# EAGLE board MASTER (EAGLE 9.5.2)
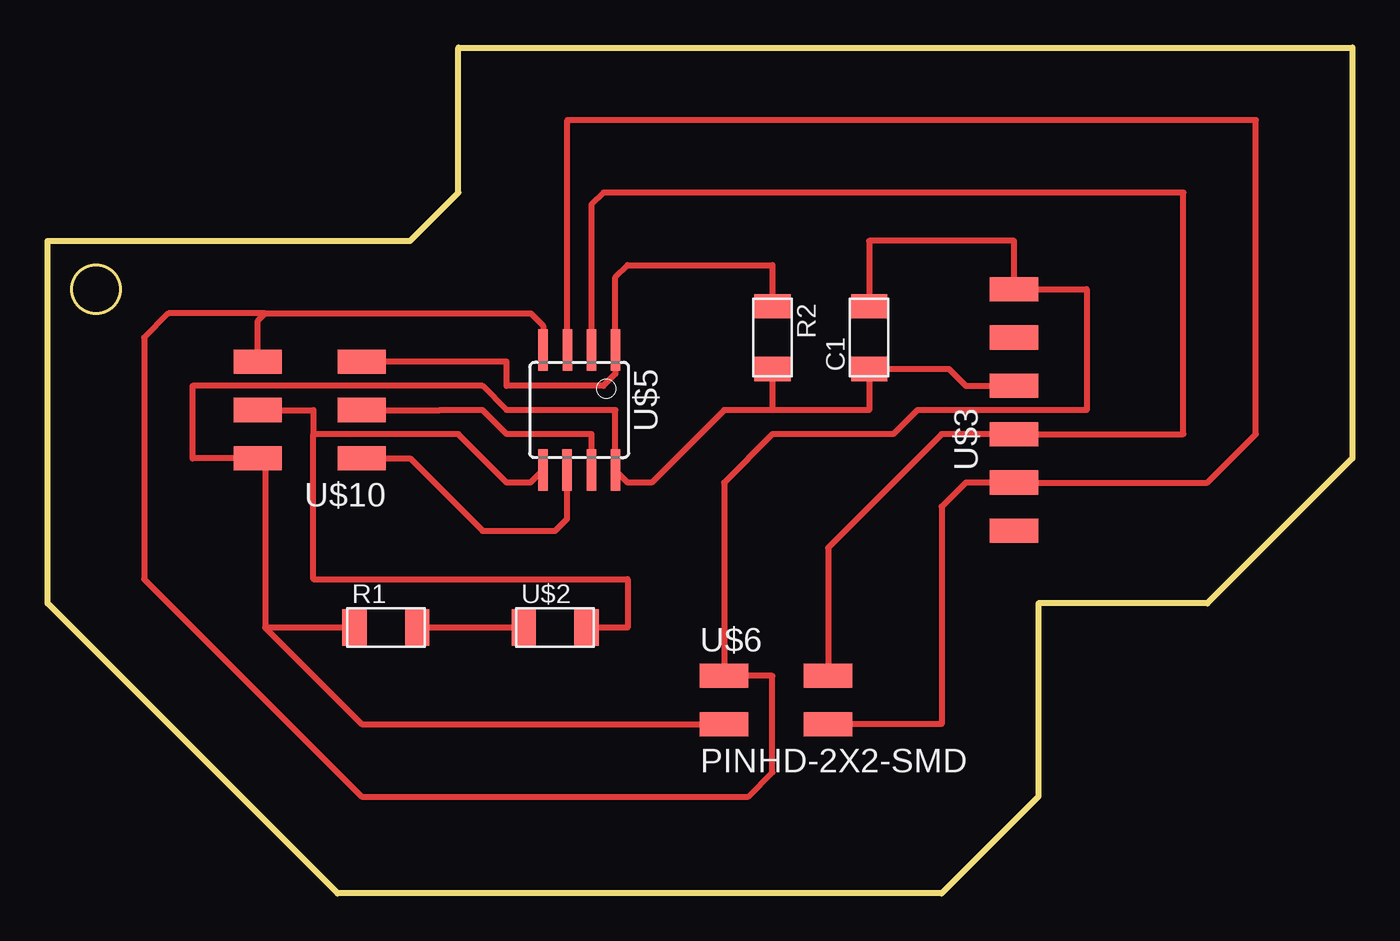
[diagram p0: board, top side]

Size 68.58 x 44.45 mm. Coordinates in mm from the lower left corner, seen from the top.
Outline: 0,34.29 19.05,34.29 21.59,36.83 21.59,44.45 68.58,44.45 68.58,22.86 60.96,15.24 52.07,15.24 52.07,5.08 46.99,0 15.24,0 0,15.24 0,34.29
Outline: circle at 2.54,31.75 radius 1.27
Copper layers (1*16): Top 0.035mm / dielectric 1.5mm / Bottom 0.035mm
Design rules "default": minimum track width 6mil, minimum drill 0.35mm, track to track 6mil, track to pad 6mil, pad to pad 6mil, via to via 6mil, smd to smd 6mil, copper to edge 40mil, drill to drill 6mil, minimum pad ring 10mil, minimum via ring 8mil, stop-mask expansion 4mil, vias tented up to drill 0mil, thermal gap 10mil

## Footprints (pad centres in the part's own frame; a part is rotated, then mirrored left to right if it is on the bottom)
C1206FAB = smd 1.27 x 1.905: 1 -1.651,0; 2 1.651,0
R1206FAB = smd 1.27 x 1.905: 1 -1.651,0; 2 1.651,0
LED1206FAB = smd 1.27 x 1.905: 1 -1.651,0; 2 1.651,0
1X06SMD = smd 2.54 x 1.27: 1 0,6.35; 2 0,3.81; 3 0,1.27; 4 0,-1.27; 5 0,-3.81; 6 0,-6.35
SOIC8 = smd 0.5 x 2.2: 1 -1.905,-3.154; 2 -0.645,-3.154; 3 0.625,-3.154; 4 1.895,-3.154; 5 1.905,3.154; 6 0.635,3.154; 7 -0.635,3.154; 8 -1.905,3.154
2X02SMD = smd 2.54 x 1.27: 1 -2.54,1.27; 2 2.92,1.27; 3 -2.54,-1.27; 4 2.92,-1.27
2X03SMD = smd 2.54 x 1.27: 1 -2.54,2.54; 2 2.92,2.54; 3 -2.54,0; 4 2.92,0; 5 -2.54,-2.54; 6 2.92,-2.54

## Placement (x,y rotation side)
C1  CAP-US1206FAB  [C1206FAB]  43.18,29.21 90 top
R1  [R1206FAB]  17.78,13.97 0 top
R2  [R1206FAB]  38.1,29.21 270 top
U$2  LEDFAB1206  [LED1206FAB]  26.67,13.97 0 top
U$3  FTDI-SMD-HEADER  [1X06SMD]  50.8,25.4 0 top
U$5  ATTINY45SI  [SOIC8]  27.94,25.4 180 top
U$6  PINHD-2X2-SMD  [2X02SMD]  38.1,10.16 0 top
U$10  AVRISPSMD  [2X03SMD]  13.97,25.4 180 top

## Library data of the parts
C1 R1 R2 U$2 U$3 U$5 U$6 U$10 = eagle_fab

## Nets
GND: C1.2 U$3.1 U$5.4 U$6.1 U$10.6
MISO: U$5.6 U$10.1
MOSI: U$2.2 U$5.5 U$10.4
N$2: R1.2 U$2.1
RST: R2.1 U$5.1 U$10.5
RXD: U$3.5 U$5.3 U$6.4
SCK: U$5.7 U$10.3
TXD: U$3.4 U$5.2 U$6.2
VCC: C1.1 R1.1 R2.2 U$3.3 U$5.8 U$6.3 U$10.2

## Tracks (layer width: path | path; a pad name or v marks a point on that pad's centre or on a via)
GND
  Top 0.152: 26.04,29.21 U$5.4
  Top 0.305: C1.2 43.18,34.29 50.8,34.29 U$3.1 54.61,31.75 54.61,25.4 45.72,25.4 44.45,24.13 38.1,24.13 35.56,21.59 U$6.1 38.1,11.43 38.1,6.35 36.83,5.08 16.51,5.08 5.08,16.51 5.08,29.21 6.35,30.48 11.43,30.48 | 11.43,30.48 25.4,30.48 26.04,29.83 26.04,29.21 | U$10.6 11.05,30.1 11.43,30.48
MISO
  Top 0.305: U$10.1 19.05,22.86 22.86,19.05 26.67,19.05 27.3,19.68 U$5.6
MOSI
  Top 0.305: U$10.4 13.97,25.4 13.97,24.13 | U$5.5 25.38,21.59 24.13,21.59 21.59,24.13 13.97,24.13 | 13.97,24.13 13.97,16.51 30.48,16.51 30.48,13.97 U$2.2
N$2
  Top 0.305: U$2.1 R1.2
RST
  Top 0.305: U$10.5 24.13,27.94 24.13,26.67 29.21,26.67 29.85,27.31 U$5.1 29.85,32.39 30.48,33.02 38.1,33.02 R2.1
RXD
  Top 0.152: 40.64,8.89 U$6.4
  Top 0.305: U$5.3 27.32,40.64 63.5,40.64 63.5,24.13 60.96,21.59 U$3.5 48.26,21.59 46.99,20.32 46.99,8.89 40.64,8.89
SCK
  Top 0.305: U$5.7 28.57,24.13 24.13,24.13 22.86,25.4 20.62,25.4 U$10.3
TXD
  Top 0.305: U$6.2 41.02,18.16 46.99,24.13 U$3.4 59.69,24.13 59.69,36.83 50.18,36.83 49.53,36.83 29.21,36.83 28.58,36.2 U$5.2
VCC
  Top 0.305: U$3.3 48.26,26.67 47.37,27.56 C1.1 43.18,25.4 38.1,25.4 | 38.1,25.4 35.56,25.4 31.75,21.59 30.48,21.59 29.85,22.22 U$5.8 29.85,25.4 24.13,25.4 22.86,26.67 7.62,26.67 7.62,22.86 U$10.2 11.43,22.48 11.43,13.97 | R2.2 38.1,25.4 | R1.1 11.43,13.97 | 11.43,13.97 16.51,8.89 U$6.3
